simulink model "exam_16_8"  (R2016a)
settings: Solver=VariableStepAuto  StartTime=0.0  StopTime=10.0  RelTol=1e-3

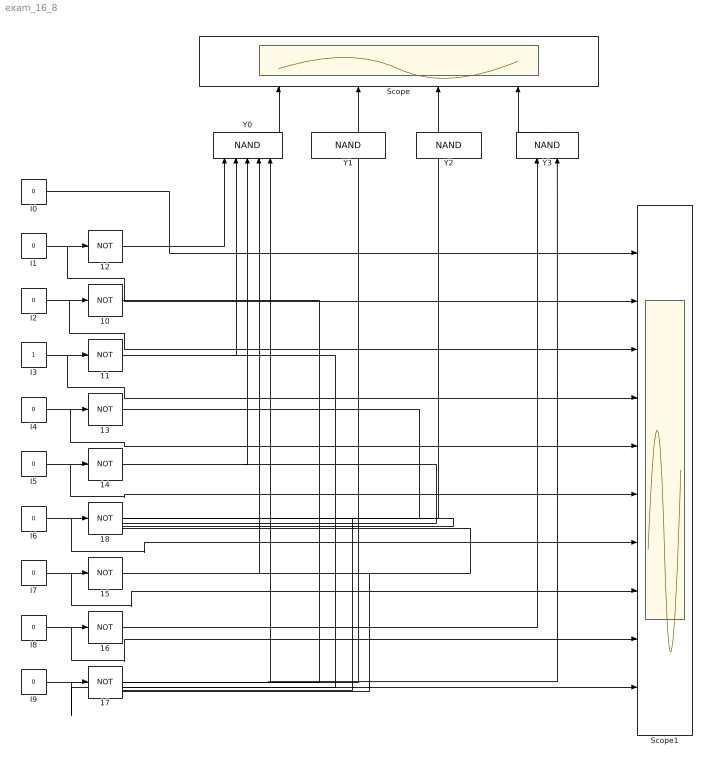
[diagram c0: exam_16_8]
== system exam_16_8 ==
  {10..18} (9 alike) : Logic  Operator=NOT  Inputs=1  AllPortsSameDT=off  OutDataTypeStr=boolean
  I{0..2,4..9} (9 alike) : Constant  Value=0
  I3 : Constant
  Scope : Scope  NumInputPorts=4
  Scope1 : Scope  NumInputPorts=10
  Y0 : Logic  Operator=NAND  Inputs=5  AllPortsSameDT=off  OutDataTypeStr=boolean
  Y1 : Logic  Operator=NAND  Inputs=4  AllPortsSameDT=off  OutDataTypeStr=boolean
  Y2 : Logic  Operator=NAND  Inputs=4  AllPortsSameDT=off  OutDataTypeStr=boolean
  Y3 : Logic  Operator=NAND  AllPortsSameDT=off  OutDataTypeStr=boolean
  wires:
  Y0/1 -> Scope/1
  Y1/1 -> Scope/2
  Y2/1 -> Scope/3
  Y3/1 -> Scope/4
  I1/1 -> Scope1/2, 12/1
  I2/1 -> Scope1/3, 11/1
  I3/1 -> Scope1/4, 12/1
  I4/1 -> Scope1/5, 13/1
  I5/1 -> Scope1/6, 14/1
  I6/1 -> Scope1/7, 18/1
  I7/1 -> Scope1/8, 15/1
  I8/1 -> Scope1/9, 16/1
  I9/1 -> Scope1/10, 17/1
  12/1 -> Y0/1
  11/1 -> Y1/1
  12/1 -> Y0/2, Y1/2
  13/1 -> Y2/1
  14/1 -> Y2/2, Y0/3
  18/1 -> Y1/3, Y2/3
  15/1 -> Y0/4, Y1/4, Y2/4
  16/1 -> Y3/1
  17/1 -> Y0/5, Y3/2
  I0/1 -> Scope1/1
